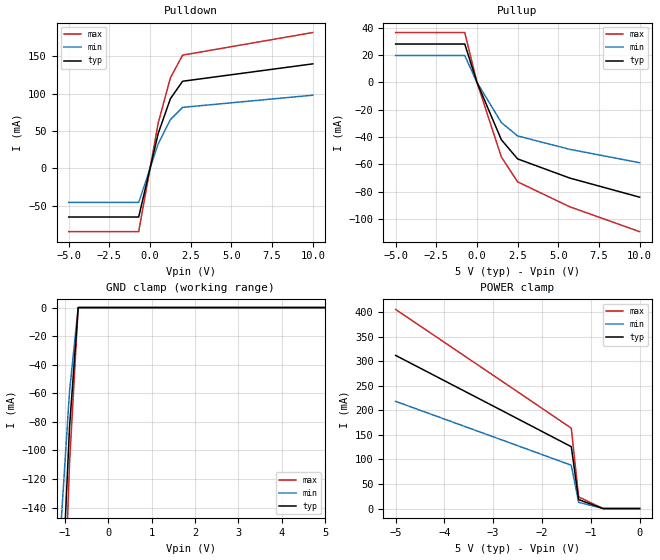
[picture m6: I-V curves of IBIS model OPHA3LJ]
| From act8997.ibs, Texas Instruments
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[Model]   OPHA3LJ
| 16-mA 3-state CMOS/TTL output buffer with 0.125 di/dt and active-low enable
| OP (97318 ALEY)
| BP (97318 ALEY)
Model_type   3-state
Polarity   Non-Inverting
| Signals   DCO (3-state)
| variable   typ   min   max
C_comp   15pF   NA   NA
| variable   typ   min   max
[Voltage range]   5.0V   4.5V   5.5V
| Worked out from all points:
|   slope of the pulldown table from 0 to 0.75 V, typ, clamps not added: 12.1 ohm
|   slope of the pullup table from 0 to 0.75 V, typ, clamps not added: 35.7 ohm
|   GND clamp passes 1 mA (typ) near -0.70 V on its own axis
[pullup]
|   50C:5V:   100C:4.5V:weak  0C:5.5V:strong
| Voltage   I(typ)   I(min)   I(max)
-5V       28mA       19.6mA     36.4mA
-2.75V    28mA       19.6mA     36.4mA
-1.4V     28mA       19.6mA     36.4mA
-1.25V    28mA       19.6mA     36.4mA
-750mV    28mA       19.6mA     36.4mA
0V        0A         0A         0A
1.5V      -42mA      -29.4mA    -54.6mA
2.5V      -56mA      -39.2mA    -72.8mA
5.7V      -70mA      -49mA      -91mA
10V       -84mA      -58.8mA    -109.2mA
[pulldown]
|   50C:5V:   100C:4.5V:weak  0C:5.5V:strong
| Voltage   I(typ)   I(min)   I(max)
-5V       -65.3mA    -45.7mA    -84.9mA
-900mV    -65.3mA    -45.7mA    -84.9mA
-700mV    -65.3mA    -45.7mA    -84.9mA
-500mV    -46.7mA    -32.7mA    -60.7mA
0V        0A         0A         0A
500mV     46.7mA     32.7mA     60.7mA
1.25V     93.3mA     65.3mA     121.3mA
2V        116.7mA    81.7mA     151.7mA
10V       140mA      98mA       182mA
[power_clamp]
|   50C:5V:   100C:4.5V:weak  0C:5.5V:strong
| Voltage   I(typ)   I(min)   I(max)
-5V       312.2mA    218.5mA    405.9mA
-2.75V    196mA      137.2mA    254.8mA
-1.4V     126mA      88.2mA     163.8mA
-1.25V    18.2mA     12.7mA     23.7mA
-750mV    0A         0A         0A
0V        0A         0A         0A
[gnd_clamp]
|   50C:5V:   100C:4.5V:weak  0C:5.5V:strong
| Voltage   I(typ)   I(min)   I(max)
-5V       -2.8A      -2A        -3.6A
-900mV    -84mA      -58.8mA    -109.2mA
-700mV    0A         0A         0A
0V        0A         0A         0A
5V        0A         0A         0A
[ramp]
| variable   typ   min   max
dV/dt_r   1.5/2.25e-9   1.2/3.375e-9   1.8/1.5e-9
dV/dt_f   2.3/3e-9   1.9/4.5e-9   2.7/2e-9
